(* Logix 5000 AddOnInstructionDefinition export CM1T_MoveRelative; software revision 20.00 *)

TYPE CM1T_DriveStatus :
STRUCT
   StatusValue : SINT;   // Indicates status and error type
   StatusValue1 : SINT;   // Additional status values
   In_Position : BOOL;   // Drive is in position and ready to move
   Moving : BOOL;   // Drive is currently moving
   Disabled : BOOL;   // Drive is disabled
   Error : BOOL;   // Drive is in an error state
   MoveComplete : BOOL;   // Move Complete
   NewStartRequired : BOOL;   // New setpoint required
   HomeAchieved : BOOL;   // Home achieved
END_STRUCT
END_TYPE

TYPE CM1T_Controlword :
STRUCT
   Start : BOOL;   // Start a motion or set a new setpoint
   Halt : BOOL;   // Halt the current motion
   Relative_Move : BOOL;   // Execute the position profile as a relative move
   Speed_Control : BOOL;   // Execute the profile as speed control only
   Disable : BOOL;   // Disable the drive (zero torque)
   Reset_Error : BOOL;   // Reset any existing errors with rising edge
   Set_to_Zero : BOOL;   // Set the current position to 0
   Home : BOOL;   // Execute a home search
END_STRUCT
END_TYPE

TYPE CM1T_Axis :
STRUCT
   Input : SINT[32];   // Data coming from the CM1-T
   Output : SINT[20];   // Data going to the CM1-T
   us50Counter : DINT;   // Controller 50us counter
   ClearCounter : BOOL;
   ModeOfOperation : SINT;   // Type of motion control mode
   ModeOfOperationDisplay : SINT;   // Indicates the active control mode
   Controlword : CM1T_Controlword;   // Controls the drive operation
   DriveStatus : CM1T_DriveStatus;   // Shows status of the drive
   PositionTarget : DINT;   // Final target position for position move
   SpeedTarget : DINT;   // Maximum speed for target move
   TorqueTarget : INT;   // Max torque allowed in 0.1% of peak. Typically 1100
   AccelerationTarget : INT;   // Acceleration for profile move
   DecelerationTarget : INT;   // Deceleration for profile move
   PositionActual : DINT;   // Actual position of the drive
   TargetActual : DINT;   // 1ms position target
   PositionError : DINT;   // Error between the current drive position and the instantaneous target position
   SpeedActual : DINT;   // Actual speed of the drive
   CurrentActual : INT;   // 0.1% of rated current
   OverloadActual : INT;   // 0.1% of overload torque
   DCVoltage : INT;   // DC voltage bus. 0.1V unit
   AnalogIN : INT;   // Value of 10bit analog input
   DigitalIN : SINT;   // Read the digital inputs
   DigitalOUT : SINT;   // Set the digital outputs
   Temperature : SINT;   // Temperature of the drive
   ErrorCode : SINT;   // Indicates error in Ethernet/IP module
END_STRUCT
END_TYPE

ADD_ON_INSTRUCTION CM1T_MoveRelative   (* revision 1.0 *)
// Relative Position Move
VAR_IN_OUT
   CM1T_Axis : CM1T_Axis; {required}
        .CONTROLWORD.RELATIVE_MOVE   // Set absolute move
END_VAR
VAR_INPUT
   Position : DINT; {required}
   Speed : DINT; {required}
   Acceleration : INT; {required}
   Deceleration : INT; {visible}
   Start : BOOL; {required}
END_VAR
VAR
   storage_Start : BOOL; {access None}
   output_Start : BOOL; {access None}
END_VAR

ROUTINE Logic   (* ladder *)
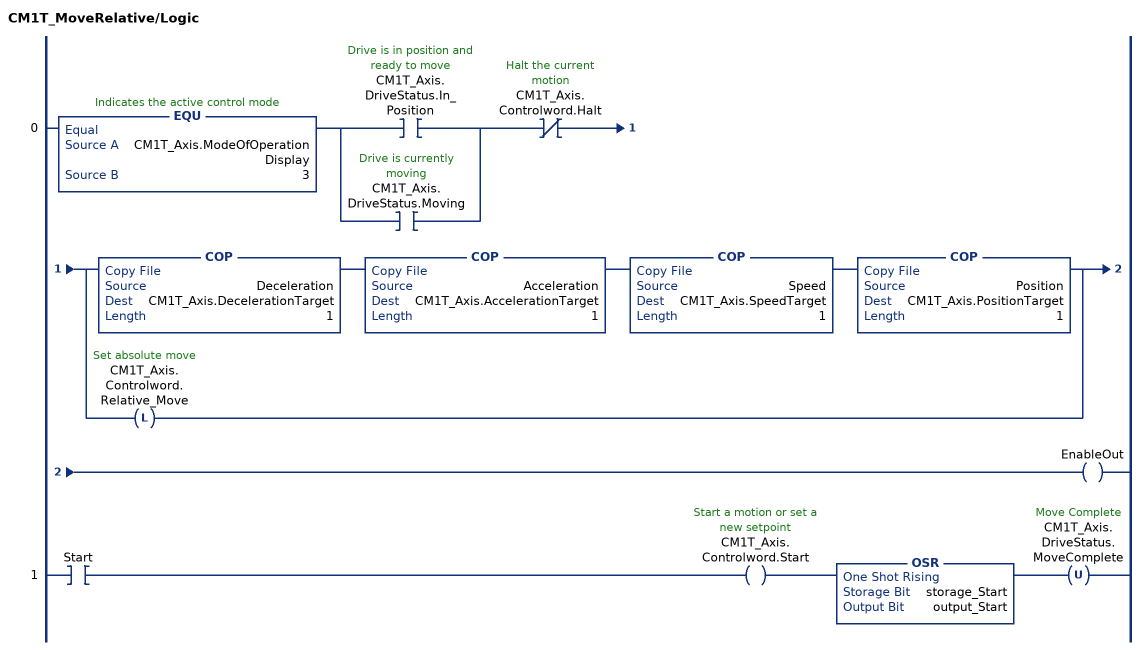
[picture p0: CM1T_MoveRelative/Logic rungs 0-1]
   0: EQU(CM1T_Axis.ModeOfOperationDisplay,3)[XIC(CM1T_Axis.DriveStatus.In_Position) ,XIC(CM1T_Axis.DriveStatus.Moving) ]XIO(CM1T_Axis.Controlword.Halt)[COP(Deceleration,CM1T_Axis.DecelerationTarget,1) COP(Acceleration,CM1T_Axis.AccelerationTarget,1) COP(Speed,CM1T_Axis.SpeedTarget,1) COP(Position,CM1T_Axis.PositionTarget,1) ,OTL(CM1T_Axis.Controlword.Relative_Move) ]OTE(EnableOut);
   1: XIC(Start)OTE(CM1T_Axis.Controlword.Start)OSR(storage_Start,output_Start)OTU(CM1T_Axis.DriveStatus.MoveComplete);
END_ROUTINE
END_ADD_ON_INSTRUCTION
